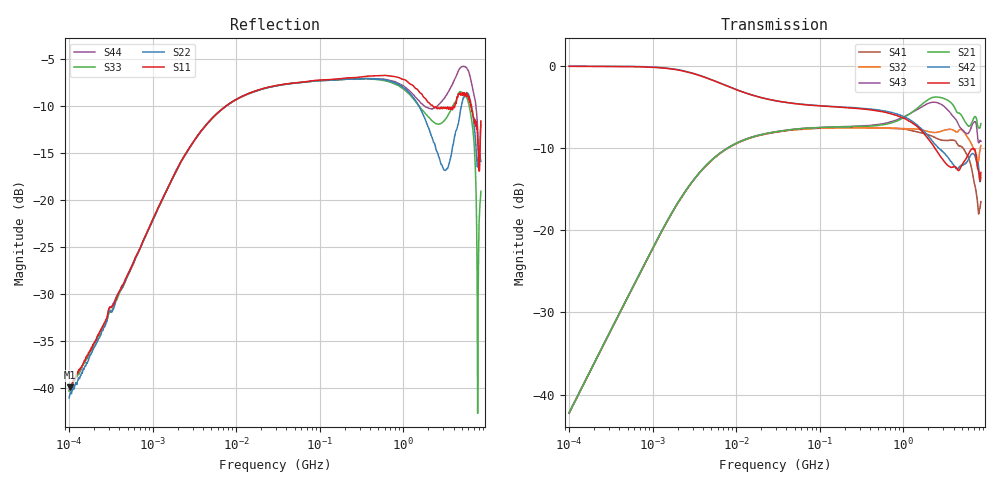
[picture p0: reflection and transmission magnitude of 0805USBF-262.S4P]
# Hz S dB R 50
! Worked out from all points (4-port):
!   801 points, 100 kHz to 8.5 GHz, reference 50 ohm
!   strongest paths, dB at 100 kHz, 1.721 MHz, 29.51 MHz, 502.3 MHz, 8.5 GHz:
!     S31: 0.0, -0.4, -4.2, -5.5, -13.0
!     S42: 0.0, -0.3, -4.2, -5.4, -13.6
!     S21: -42.2, -17.8, -8.0, -7.2, -7.0
!     S43: -42.2, -17.8, -8.0, -7.1, -9.2
!     S32: -42.2, -17.8, -8.1, -7.6, -9.7
!     S41: -42.3, -17.8, -8.1, -7.5, -16.5
!   lowest |S11| = -39.9 dB at 101.7 kHz (marker M1), VSWR 1.02, Z = 50.3 + j0.986 ohm
!   |S11| at or under -10 dB: start of sweep to 7.52 MHz; 2.277 GHz to 4.135 GHz (1.858 GHz wide, 58 % of centre); 6.554 GHz to end of sweep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
100000  -39.74 75.3  -42.16 88.3  -0.05 -0.5  -42.26 -92.1
        -42.22 88.0  -41.02 70.2  -42.29 -91.5  -0.03 -0.4
        -0.05 -0.5  -42.19 -91.8  -40.31 60.7  -42.20 88.0
        -42.29 -92.1  -0.03 -0.4  -42.24 88.2  -40.20 75.4
101665  -39.87 74.9  -41.98 88.3  -0.05 -0.5  -42.10 -91.7
        -42.06 88.1  -40.77 69.8  -42.12 -92.0  -0.03 -0.4
        -0.05 -0.5  -42.10 -91.5  -40.02 61.1  -42.09 88.1
        -42.15 -92.1  -0.03 -0.4  -42.07 88.4  -40.25 76.2
1.280344e7  -8.81 22.4  -8.92 22.2  -3.27 -14.9  -8.98 -158.6
            -8.96 22.3  -8.81 22.1  -9.02 -158.6  -3.25 -14.9
            -3.28 -14.9  -8.99 -158.7  -8.82 22.2  -8.96 22.3
            -8.97 -158.7  -3.27 -15.0  -8.93 22.2  -8.85 22.5
7.175618e8  -6.80 -110.7  -6.94 -102.0  -5.81 -143.0  -7.59 35.3
            -6.94 -102.0  -7.38 -116.2  -7.61 30.9  -5.65 -141.6
            -5.83 -143.1  -7.61 31.0  -7.49 -112.0  -6.79 -104.2
            -7.56 35.4  -5.65 -141.7  -6.78 -104.1  -7.30 -110.9
1.823651e9  -9.17 57.5  -4.38 85.2  -8.38 3.0  -8.27 175.6
            -4.37 85.1  -11.35 50.9  -7.90 168.0  -8.08 6.9
            -8.38 2.7  -7.89 168.0  -10.75 65.2  -4.75 78.5
            -8.26 175.7  -8.09 6.6  -4.75 78.5  -10.05 67.6
2.843154e9  -10.11 -99.2  -3.87 -87.6  -11.12 169.3  -9.02 -17.3
            -3.86 -87.7  -16.19 -101.3  -7.95 -22.4  -10.23 176.4
            -11.13 168.7  -7.94 -22.4  -11.84 -90.3  -4.67 -95.4
            -9.02 -17.1  -10.25 175.9  -4.67 -95.4  -9.58 -89.6
8.5e9  -11.59 54.6  -7.00 95.5  -12.84 167.4  -16.90 31.8
       -7.02 95.3  -15.88 74.6  -9.76 52.4  -13.56 173.9
       -12.97 166.7  -9.70 53.2  -19.06 107.8  -9.15 77.1
       -16.52 33.2  -13.60 173.4  -9.16 76.6  -11.95 67.5
